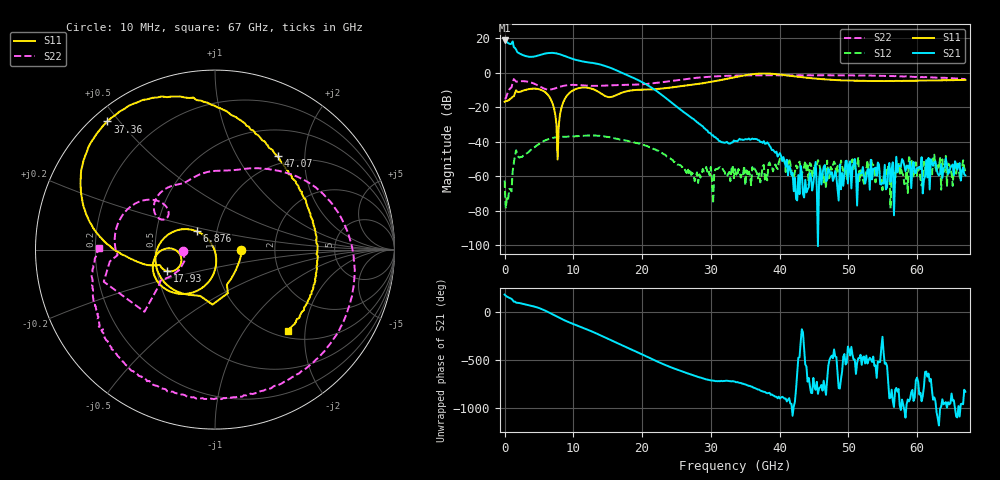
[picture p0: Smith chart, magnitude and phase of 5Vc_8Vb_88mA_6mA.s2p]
! MARKI MICROWAVE INC.
! Date:  05/05/2020
! Model Number:  APM-7099CH
! Description:  2-port Small Signal S-parameter data for APM-7099CH
! Frequency Range:  10 MHz to 67 GHz
! Port Configuration:  PORT 1: Input
!  PORT 2: Output
! Bias Condition: Vc = +5V, Vb = +8V
! APM-7099CH s2p files are only valid for small signal conditions (below -5 dBm input power)
!S2P File: Measurements: Mag<S11> Ang<S11>, Mag<S21> Ang<S21>, Mag<S12> Ang<S12>, Mag<S22> Ang<S22>!row 1
# Hz S  dB  R 50
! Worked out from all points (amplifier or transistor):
!   401 points, 10 MHz to 67 GHz, reference 50 ohm
!   highest |S21| = 18.5 dB at 10 MHz (marker M1)
!   |S21| within 3 dB of that: start of sweep to 1.304 GHz
!   unconditionally stable (mu >= 1): start of sweep to end of sweep
!   at 11.06 GHz: K = 11.51, MAG = 8.1 dB, |S12| = -36.8 dB
!   at 33.51 GHz: K = 4615.45, MAG = -31.5 dB, |S12| = -55.9 dB
!   at 67 GHz: K = 127663.47, MAG = -55.2 dB, |S12| = -57.3 dB
!   S11 on the Smith chart (normalised r, x): 10 MHz: 1.34, -0.00; 6.876 GHz: 0.80, +0.17; 17.93 GHz: 0.57, -0.15; 37.36 GHz: 0.04, +0.47; 47.07 GHz: 0.88, +1.50; 67 GHz: 1.12, -1.63
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1e7  -16.86 -0.5  18.55 177.8  -62.54 20.4  -14.85 -178.0
1.01485e9  -14.66 -60.5  16.70 133.1  -68.78 -4.9  -8.55 -147.1
1.3498e9  -13.71 -71.3  14.64 103.3  -52.19 -26.5  -3.81 -163.9
1.68475e9  -10.27 -92.6  13.24 94.0  -44.98 -88.6  -5.29 -176.8
2.35465e9  -11.00 -115.5  10.67 86.4  -48.82 -133.6  -5.00 173.8
5.201725e9  -9.86 179.1  10.21 32.8  -40.75 143.4  -8.22 138.5
6.876475e9  -16.79 135.0  11.36 -23.2  -38.00 87.5  -9.70 149.1
7.71385e9  -50.36 -173.2  10.87 -54.5  -37.41 61.6  -8.68 150.6
8.38375e9  -18.87 -90.1  10.10 -78.3  -37.15 42.0  -7.88 147.3
9.72355e9  -10.91 -120.9  8.11 -120.0  -36.95 6.8  -7.16 135.5
1.123082e10  -8.74 -149.5  6.51 -161.7  -36.64 -30.8  -7.38 123.6
1.424538e10  -12.68 179.2  4.24 104.6  -36.80 -113.5  -7.64 109.2
1.60876e10  -13.34 -155.4  1.61 43.2  -38.21 -165.6  -7.31 98.8
1.792982e10  -10.69 -155.8  -1.69 -15.6  -39.59 145.1  -7.13 87.4
2.245165e10  -9.43 -164.9  -11.72 -164.2  -45.40 26.7  -5.81 62.3
3.3505e10  -2.69 165.6  -39.62 -5.6  -55.86 15.8  -1.78 -25.3
3.735692e10  -0.61 130.0  -40.13 -101.8  -59.37 21.1  -1.58 -51.8
4.22137e10  -2.22 85.3  -60.95 146.0  -57.42 -122.8  -1.61 -77.9
4.472582e10  -3.33 69.5  -68.25 -124.4  -59.60 -97.7  -1.62 -89.7
4.707048e10  -4.07 56.1  -55.60 159.5  -61.25 -119.9  -1.57 -100.4
5.594665e10  -4.87 7.2  -52.32 -177.9  -55.58 132.4  -2.01 -136.6
6.7e10  -4.30 -48.2  -59.57 -110.3  -57.34 -64.3  -3.77 179.0
